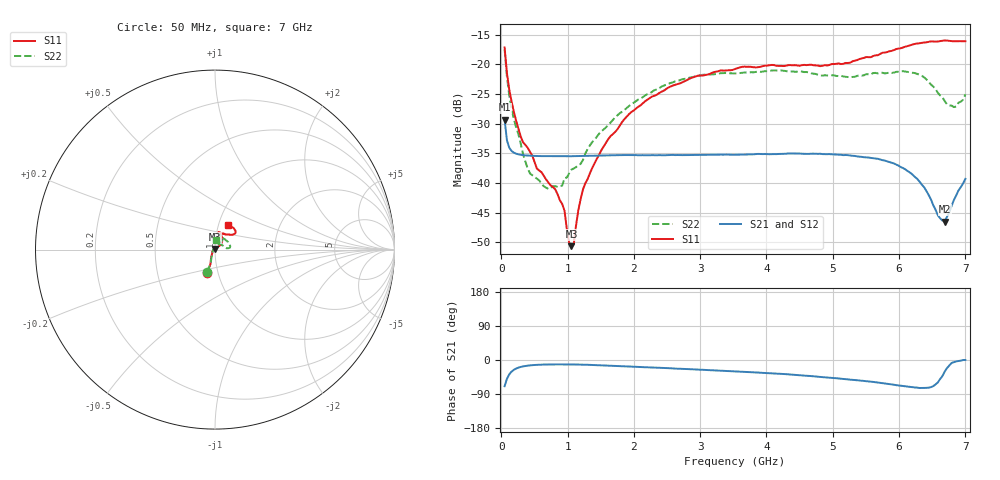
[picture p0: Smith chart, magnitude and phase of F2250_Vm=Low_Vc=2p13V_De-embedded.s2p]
! Integrated Device Technology
! Corporate Headquarters
! 6024 Silver Creek Valley Road
! San Jose, CA 95138  USA
! Phone:  1-408-284-8200
! Toll Free:  1-800-223-1366
! Webpage:  http://www.idt.com/
! Timing and RF Division
! 515 Groton Road, Suite 102
! Westford, MA 01886-6024
! Device:  F2250
! Description: Voltage Variable RF Attenuator
! Frequency:  50.0 -  6000.00 MHz
! Package:  3x3 mm Thin QFN Plastic Package: 16 pin
! Ports:  2 RF, 3 DC
!  Pin  1  = GND
!  Pin  2  = NC
!  Pin  3  = RF1  = Port 1
!  Pin  4  = NC
!  Pin  5  = GND
!  Pin  6  = GND
!  Pin  7  = GND
!  Pin  8  = GND
!  Pin  9  = NC
!  Pin 10  = RF2  = Port 2
!  Pin 11  = NC
!  Pin 12  = GND
!  Pin 13  = GND
!  Pin 14  = VCNTRL
!  Pin 15  = VDD
!  Pin 16  = VMODE
! Vcntrl:  2.130 Volts
! Vmode:  +0.000 Volts
! Vdd:  +3.30  Volts
! Current:  1.181 mA
! Data:  The device was measured on a the F2250 evaluation board which has
!  individual transmission lines to the RF pins.  Data was collected
!  using a calibrated network analyzer.  The evaluation board was
!  de-embedded using a TRL calibration technique.
!  The reference plane is the edge of the package pin.
! Misc:  SN 10
!  Action Tracker AT0258
! Date Measured:  2014-11-26
! Date:  2015-10-15  MJV
! Note:
!  Integrated Device Technology supplies this data as a sample of measured
!  data at the package pin for this product.  Your particular data for this
!  product may vary.
!  Data was taken at 25 degrees C.
!  Integrated Device Technology reserves the right to change this data at anytime.
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# GHz S dB R 50
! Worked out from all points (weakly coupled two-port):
!   201 points, 50 MHz to 7 GHz, reference 50 ohm
!   highest |S21| = -29.35 dB at 50 MHz (marker M1); lowest = -46.5 dB at 6.687 GHz (marker M2)
!   lowest |S11| = -50.7 dB at 1.058 GHz (marker M3), VSWR 1.01, Z = 49.8 + j0.245 ohm
!   |S11| at or under -10 dB: start of sweep to end of sweep
!   |S22| runs from -41.0 to -17.5 dB; largest |S21 - S12| = 5.7e-05
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0.05  -17.18 -108.6  -29.35 -69.1  -29.35 -69.1  -17.50 -109.9
0.08475  -21.45 -107.4  -32.81 -49.8  -32.81 -49.7  -22.07 -107.6
0.189  -28.00 -119.6  -34.90 -25.9  -34.90 -25.9  -29.26 -120.8
0.328  -33.16 -133.8  -35.32 -16.9  -35.32 -16.9  -35.15 -135.8
0.43225  -34.72 -144.6  -35.42 -14.2  -35.42 -14.2  -38.40 -161.6
0.71025  -39.94 -168.3  -35.50 -11.8  -35.51 -11.8  -41.03 149.1
0.91875  -43.56 157.9  -35.52 -11.6  -35.52 -11.6  -40.45 117.5
0.9535  -44.69 169.7  -35.52 -11.6  -35.52 -11.6  -39.18 116.9
1.023  -50.08 144.0  -35.50 -11.7  -35.51 -11.7  -38.39 98.1
1.05775  -50.67 122.8  -35.50 -11.7  -35.50 -11.7  -37.75 93.4
1.0925  -50.41 90.4  -35.49 -11.8  -35.49 -11.8  -37.57 88.5
1.162  -44.61 56.8  -35.47 -12.0  -35.47 -12.0  -37.00 77.3
1.2315  -41.12 44.2  -35.44 -12.2  -35.44 -12.2  -36.14 68.4
1.6485  -32.11 41.9  -35.36 -14.8  -35.36 -14.8  -29.84 56.0
2.37825  -24.88 47.3  -35.32 -20.6  -35.32 -20.6  -24.06 52.5
3.525  -20.80 72.5  -35.26 -29.9  -35.26 -29.9  -21.55 72.6
4.7065  -20.17 72.4  -35.07 -43.0  -35.07 -43.0  -21.59 71.0
5.85325  -17.82 40.4  -36.48 -63.6  -36.49 -63.7  -21.42 20.7
6.33975  -16.41 41.0  -40.26 -73.8  -40.25 -73.8  -21.93 6.6
6.68725  -15.99 48.8  -46.51 -30.7  -46.48 -30.3  -26.19 26.6
6.861  -16.12 55.1  -42.12 -3.7  -42.08 -3.5  -27.11 58.2
7  -16.12 63.2  -39.32 0.0  -39.28 -0.1  -25.08 84.8
